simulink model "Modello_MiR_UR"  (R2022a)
settings: Solver=FixedStepAuto  StartTime=0.0  StopTime=time_s(end,1)  FixedStep=Sim.dt*10  RelTol=1e-3  EnableMultiTasking=on
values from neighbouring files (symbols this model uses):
  a = 0.250    (= 0.25)    [Modello_MiR_UR_script.m]    (also in Modello_MiR_2ruote_script.m; Modello_MiR_6ruote_script.m; Modello_MiR_6ruote_validato_script.m)
  a1 = 0.18265    [Modello_MiR_UR_script.m]    (also in UR_DHtable_e.m = 0; Modello_MiR_2ruote_script.m = deg2rad(5); Modello_MiR_6ruote_script.m = deg2rad(5); Modello_MiR_6ruote_validato_script.m)
  a2 = 0.40857    [Modello_MiR_UR_script.m]    (also in UR_DHtable_e.m = 612; Modello_MiR_2ruote_script.m = deg2rad(25); Modello_MiR_6ruote_script.m = deg2rad(25); Modello_MiR_6ruote_validato_script.m)
  Att_C1 = 0.01    [Modello_MiR_UR_script.m]    (also in Modello_MiR_6ruote_validato_script.m)
  Att_C2 = 0.01    [Modello_MiR_UR_script.m]    (also in Modello_MiR_6ruote_validato_script.m)
  Att_C5 = 0.01    [Modello_MiR_UR_script.m]    (also in Modello_MiR_6ruote_validato_script.m)
  Att_C6 = 0.01    [Modello_MiR_UR_script.m]    (also in Modello_MiR_6ruote_validato_script.m)
  b = 0.1875    [Modello_MiR_UR_script.m]    (also in Modello_MiR_2ruote_script.m; Modello_MiR_6ruote_script.m; Modello_MiR_6ruote_validato_script.m)
  b_caster = 0.07    [Modello_MiR_UR_script.m]    (also in Modello_MiR_2ruote_script.m; Modello_MiR_6ruote_script.m; Modello_MiR_6ruote_validato_script.m)
  bd = 0.205    [Modello_MiR_UR_script.m]    (also in Modello_MiR_2ruote_script.m; Modello_MiR_6ruote_script.m; Modello_MiR_6ruote_validato_script.m)
  F23MIR = @(u) (mv*9.801/4)-(mv*h*u(5)+(mv*9.801/4)*(2*a-b_caster*(cos(u(1))+cos(u(2)))))/(4*a-b_caster*(cos(u(1))+cos(u(2)))+b_caster*(cos(u(3))+cos(u(4))))    [Modello_MiR_UR_script.m]
  F23UR5 = @(u) (u(7)/4)-u(11)    [Modello_MiR_UR_script.m]
  F43MIR = @(u) (1/(2*bd))*(mv*u(6)*h+((mv*h*u(5)+(mv*9.801/4)*(2*a-b_caster*(cos(u(1))+cos(u(2)))))/(4*a-b_caster*(cos(u(1))+cos(u(2)))+b_caster*(cos(u(3))+cos(u(4)))))*(2*bd-b_caster*(sin(u(3))+sin(u(4))))+((mv*9.801/4)-(mv*h*u(5)+(mv*9.801/4)*(2*a-b_caster*(cos(u(1))+cos(u(2)))))/(4*a-b_caster*(cos(u(1))+cos(u(2)))+b_caster*(cos(u(3))+cos(u(4)))))*(2*bd-b_caster*(sin(u(1))+sin(u(2)))))    [Modello_MiR_UR_script.m]
  F43UR5 = @(u) (1/(2*bd))*(u(8) - u(6)*H +u(11)*(2*bd-b_caster*(sin(u(3))+sin(u(4))))+u(12)*(2*bd-b_caster*(sin(u(1))+sin(u(2)))))    [Modello_MiR_UR_script.m]
  F63MIR = @(u) (mv*h*u(5)+(mv*9.801/4)*(2*a-b_caster*(cos(u(1))+cos(u(2)))))/(4*a-b_caster*(cos(u(1))+cos(u(2)))+b_caster*(cos(u(3))+cos(u(4))))    [Modello_MiR_UR_script.m]
  F63UR5 = @(u)(-a*u(7)/2 -u(5)*H -u(9) +(u(7)/4)*(2*a-b_caster*(cos(u(1))+cos(u(2)))))/(4*a-b_caster*(cos(u(1))+cos(u(2)))+b_caster*(cos(u(3))+cos(u(4))))    [Modello_MiR_UR_script.m]
  f_c = 0.29564    [Modello_MiR_UR_script.m]    (also in Modello_MiR_6ruote_validato_script.m)
  f_d3 = 0.35846    [Modello_MiR_UR_script.m]    (also in Modello_MiR_6ruote_validato_script.m)
  f_d4 = 0.2333    [Modello_MiR_UR_script.m]    (also in Modello_MiR_6ruote_validato_script.m)
  fa_c = 0.27474    [Modello_MiR_UR_script.m]    (also in Modello_MiR_6ruote_validato_script.m)
  fa_d3 = 0.3694    [Modello_MiR_UR_script.m]    (also in Modello_MiR_6ruote_validato_script.m)
  fa_d4 = 0.28065    [Modello_MiR_UR_script.m]    (also in Modello_MiR_6ruote_validato_script.m)
  fm_fun = @(u) (u <= -am2 || u >= am2) * 0 + (u > -am2 && u <= -am1) * (- u* Mza/(am2 -am1) - Mza* am2/(am2 -am1)) +           + (u > -am1 && u <= am1) * (Mza * u / am1) + (u > am1 && u < am2) * (Mza * u /(am1 -am2) - Mza * am2 /(am1 - am2))    [Modello_MiR_UR_script.m]    (also in Modello_MiR_6ruote_script.m = @(u) (u <= -am2 | u >= am2)*0 + (u > -am2 && u <= -am1)*(- u; Modello_MiR_6ruote_validato_script.m)
  Hi = 1    [UR5e_data.m]
  Icw_1 = 1/2 * mcw * rc^2    (= 0.002004225735)    [Modello_MiR_UR_script.m]    (also in Modello_MiR_2ruote_script.m; Modello_MiR_6ruote_script.m; Modello_MiR_6ruote_validato_script.m)
  Icw_2 = 1/12 * mcw * ec^2 + 1/4 * mcw * rc^2    (= 0.00104098243873)    [Modello_MiR_UR_script.m]    (also in Modello_MiR_2ruote_script.m; Modello_MiR_6ruote_script.m; Modello_MiR_6ruote_validato_script.m)
  Idw_1 = 1/2 * mdw * rd^2    (= 0.00551836278784)    [Modello_MiR_UR_script.m]    (also in Modello_MiR_2ruote_script.m; Transfer_Function_Gol_Gcl.m = Inertia_vect(jj,1); Modello_MiR_6ruote_script.m; Modello_MiR_6ruote_validato_script.m)
  iMax = 20.7*1.1    (= 22.77)    [Modello_MiR_UR_script.m]    (also in Modello_MiR_2ruote_script.m; Modello_MiR_6ruote_script.m; Modello_MiR_6ruote_validato_script.m)
  Iv = mv * (l^2 + w^2)  / 12    (= 6.75343333333)    [Modello_MiR_UR_script.m]    (also in Modello_MiR_2ruote_script.m; Modello_MiR_6ruote_script.m; Modello_MiR_6ruote_validato_script.m = 8.95033333333)
  Kc = 0.15    [Modello_MiR_UR_script.m]    (also in Modello_MiR_2ruote_script.m; Modello_MiR_6ruote_script.m; Modello_MiR_6ruote_validato_script.m)
  Ki_i = 1    [Modello_MiR_UR_script.m]    (also in Modello_MiR_2ruote_script.m; Modello_MiR_6ruote_script.m; Modello_MiR_6ruote_validato_script.m)
  Ki_v = 1    [Modello_MiR_UR_script.m]    (also in Modello_MiR_2ruote_script.m; Modello_MiR_6ruote_script.m; Modello_MiR_6ruote_validato_script.m)
  kk = 0.00005    (= 5e-05)    [Modello_MiR_UR_script.m]    (also in Modello_MiR_2ruote_script.m; Modello_MiR_6ruote_script.m; Modello_MiR_6ruote_validato_script.m)
  Kp_i = 5    [Modello_MiR_UR_script.m]    (also in Modello_MiR_2ruote_script.m; Modello_MiR_6ruote_script.m; Modello_MiR_6ruote_validato_script.m)
  Kp_v = 5    [Modello_MiR_UR_script.m]    (also in Modello_MiR_2ruote_script.m; Modello_MiR_6ruote_script.m; Modello_MiR_6ruote_validato_script.m)
  kv = 1.5e-6    (= 1.5e-06)    [Modello_MiR_UR_script.m]    (also in Modello_MiR_2ruote_script.m; Modello_MiR_6ruote_script.m; Modello_MiR_6ruote_validato_script.m)
  L = R * tauE    (= 0.00181134822805)    [Modello_MiR_UR_script.m]    (also in Modello_MiR_2ruote_script.m; Modello_MiR_6ruote_script.m; Modello_MiR_6ruote_validato_script.m)
  mcw = rc^2 * pi * ec * rhopoliu + 1    (= 1.02616357632)    [Modello_MiR_UR_script.m]    (also in Modello_MiR_2ruote_script.m; Modello_MiR_6ruote_script.m; Modello_MiR_6ruote_validato_script.m)
  mv = 83    [Modello_MiR_UR_script.m]    (also in Modello_MiR_2ruote_script.m; Modello_MiR_6ruote_script.m; Modello_MiR_6ruote_validato_script.m = 110)
  Phi1_start = psi_mir(1,1)    [Modello_MiR_UR_script.m]    (also in Modello_MiR_6ruote_validato_script.m)
  Phi2_start = psi_mir(1,1)    [Modello_MiR_UR_script.m]    (also in Modello_MiR_6ruote_validato_script.m)
  Phi5_start = psi_mir(1,1)    [Modello_MiR_UR_script.m]    (also in Modello_MiR_6ruote_validato_script.m)
  Phi6_start = psi_mir(1,1)    [Modello_MiR_UR_script.m]    (also in Modello_MiR_6ruote_validato_script.m)
  Psi_start = psi_mir(1,1)    [Modello_MiR_UR_script.m]    (also in Modello_MiR_6ruote_script.m = 1.57079632679; Modello_MiR_6ruote_validato_script.m)
  q0 = [qset.q1.signals.values(1),qset.q2.signals.values(1),qset.q3.signals.values(1),qset.q4.signals.values(1),qset.q5.signals.values(1),qset.q6.signals.values(1)]    [UR5e_simmot.m]
  R = velMax * TorqueMax / (iMax)^2    (= 1.81134822805)    [Modello_MiR_UR_script.m]    (also in Modello_MiR_2ruote_script.m; Modello_MiR_6ruote_script.m; Modello_MiR_6ruote_validato_script.m)
  rap_rid = 10.167    [Modello_MiR_UR_script.m]    (also in Modello_MiR_2ruote_script.m; Modello_MiR_6ruote_script.m; Modello_MiR_6ruote_validato_script.m)
  rc = 0.125/2    (= 0.0625)    [Modello_MiR_UR_script.m]    (also in Modello_MiR_2ruote_script.m; Modello_MiR_6ruote_script.m; Modello_MiR_6ruote_validato_script.m)
  rd = 0.1    [Modello_MiR_UR_script.m]    (also in Modello_MiR_2ruote_script.m; Modello_MiR_6ruote_script.m; Modello_MiR_6ruote_validato_script.m)
  s = 1i*s    [Transfer_Function_Gol_Gcl.m]
  s1 = 0.18987    [Modello_MiR_UR_script.m]    (also in Modello_MiR_2ruote_script.m = 0.2; Modello_MiR_6ruote_script.m = 0.2; Modello_MiR_6ruote_validato_script.m)
  s2 = 0.99533    [Modello_MiR_UR_script.m]    (also in Modello_MiR_2ruote_script.m = 0.8; Modello_MiR_6ruote_script.m = 0.8; Modello_MiR_6ruote_validato_script.m)
  Sx = spline(x ,fl_fun(x),zx)    [Modello_MiR_6ruote_script.m]
  Sy = spline(x ,ft_fun(x),zy)    [Modello_MiR_6ruote_script.m]
  tau_i = 1/(2000*2*pi)    (= 7.95774715459e-05)    [UR5e_data.m]    (also in Transfer_Function_Gol_Gcl.m = Kp_i/Ki_i)
  VaMax = Kc * velMax    (= 41.2443991527)    [Modello_MiR_UR_script.m]    (also in Modello_MiR_2ruote_script.m; Modello_MiR_6ruote_script.m; Modello_MiR_6ruote_validato_script.m)
  X_start = traj(1,1)    [Modello_MiR_UR_script.m]    (also in Modello_MiR_2ruote_script.m = input('Inserire coordinata x iniziale'); Modello_MiR_6ruote_script.m = input('Inserire coordinata x iniziale'); Modello_MiR_6ruote_validato_script.m)
  Y_start = traj(1,2)    [Modello_MiR_UR_script.m]    (also in Modello_MiR_2ruote_script.m = input('Inserire coordinata y iniziale'); Modello_MiR_6ruote_script.m = input('Inserire coordinata y iniziale'); Modello_MiR_6ruote_validato_script.m)
undefined symbols (not defined in the file or in its folder): deg, Driver1, Driver2, Driver3, Driver4, Driver5, Driver6, Ground, J1, J2, J3, J4, J5, J6, kg, L1, L2, L3, L4, L5, L6, m, Motor, N, X, Y, z, Z
libraries: sm_lib x33, nesl_utility x30, slpidlib x10
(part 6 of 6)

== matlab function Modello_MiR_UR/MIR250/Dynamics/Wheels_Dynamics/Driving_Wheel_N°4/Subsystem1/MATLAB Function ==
function [Sx, z] = fcn(f, fa, s1, s2)
FLa =  fa  ;
FL = f  ;
Fx = @(u) (u <= -s2).* (-FL) + (u > -s2 & u <= -s1).*(u*(FL - FLa)/(s2 - s1) + s2*(FL - FLa)/(s2 - s1) - FL) +...
        + (u > -s1 & u <= s1).*(u * FLa / s1) + (u > s1 & u <= s2).* (u * (FLa - FL)/(s1 - s2) - s2 * (FLa - FL)/(s1 - s2) + FL) + ...
        + (u> s2) * FL;
% Interpolazione Cubica Attrito Longitudinale
nvet = 23 ; %specificare i numeri di nodi ( −1) della partizione
inferior = -1; % estremo inferiore intervallo
superi = 1 ; % estremo superiore intervallo
z = linspace(inferior,superi,10001); % definisco la griglia fine su cui valutare la spline
%figure
%set(gcf,'Position',[381 175 1208 753])

n = nvet ;
x = linspace(inferior, superi, n+1); % in questo esercizio definisco i nodi di interpolazione tra loro equispaziati
Sx = spline(x ,Fx(x),z) ; % valuto la spline cubica interpolante

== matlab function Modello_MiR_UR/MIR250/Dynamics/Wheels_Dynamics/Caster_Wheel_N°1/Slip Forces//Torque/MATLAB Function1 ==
function [Sy, z] = fcn(f, fa, a1, a2)
FTa = 1200/2500/0.6 * fa;
FT = 1200/2500/0.6 * f;
Fy_D = @(u) (u <= -a2).*(-FT) + (u > -a2 & u <= -a1).* (u*(FT - FTa)/(a2 - a1) + a2*(FT - FTa)/(a2 - a1) - FT) +...
+ (u > -a1 & u <= a1).* (u * FTa / a1) + (u > a1 & u <= a2).* (u * (FTa - FT)/(a1 - a2) - a2 * (FTa - FT)/(a1 - a2) + FT) + ...
+ (u > a2).* FT;

nvet = 20 ; %specificare i numeri di nodi ( −1) della partizione
inferior = -pi/2; % estremo inferiore intervallo
superi = pi/2 ; % estremo superiore intervallo
z = linspace(inferior,superi,10001); % definisco la griglia fine su cui valutare la spline

n = nvet ;
x = linspace(inferior, superi, n+1); % in questo esercizio definisco i nodi di interpolazione tra loro equispaziati
Sy = spline(x ,Fy_D(x),z) ; % valuto la spline cubica interpolante

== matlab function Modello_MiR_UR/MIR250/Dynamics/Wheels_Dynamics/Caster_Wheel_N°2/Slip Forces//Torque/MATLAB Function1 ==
function [Sy, z] = fcn(f, fa, a1, a2)
FTa = 1200/2500/0.6 * fa;
FT = 1200/2500/0.6 * f;
Fy_D = @(u) (u <= -a2).*(-FT) + (u > -a2 & u <= -a1).* (u*(FT - FTa)/(a2 - a1) + a2*(FT - FTa)/(a2 - a1) - FT) +...
+ (u > -a1 & u <= a1).* (u * FTa / a1) + (u > a1 & u <= a2).* (u * (FTa - FT)/(a1 - a2) - a2 * (FTa - FT)/(a1 - a2) + FT) + ...
+ (u > a2).* FT;

nvet = 20 ; %specificare i numeri di nodi ( −1) della partizione
inferior = -pi/2; % estremo inferiore intervallo
superi = pi/2 ; % estremo superiore intervallo
z = linspace(inferior,superi,10001); % definisco la griglia fine su cui valutare la spline

n = nvet ;
x = linspace(inferior, superi, n+1); % in questo esercizio definisco i nodi di interpolazione tra loro equispaziati
Sy = spline(x ,Fy_D(x),z) ; % valuto la spline cubica interpolante

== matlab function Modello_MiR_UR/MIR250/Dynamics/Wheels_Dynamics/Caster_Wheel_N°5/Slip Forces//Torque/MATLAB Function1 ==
function [Sy, z] = fcn(f, fa, a1, a2)
FTa = 1200/2500/0.6 * fa;
FT = 1200/2500/0.6 * f;
Fy_D = @(u) (u <= -a2).*(-FT) + (u > -a2 & u <= -a1).* (u*(FT - FTa)/(a2 - a1) + a2*(FT - FTa)/(a2 - a1) - FT) +...
+ (u > -a1 & u <= a1).* (u * FTa / a1) + (u > a1 & u <= a2).* (u * (FTa - FT)/(a1 - a2) - a2 * (FTa - FT)/(a1 - a2) + FT) + ...
+ (u > a2).* FT;

nvet = 20 ; %specificare i numeri di nodi ( −1) della partizione
inferior = -pi/2; % estremo inferiore intervallo
superi = pi/2 ; % estremo superiore intervallo
z = linspace(inferior,superi,10001); % definisco la griglia fine su cui valutare la spline

n = nvet ;
x = linspace(inferior, superi, n+1); % in questo esercizio definisco i nodi di interpolazione tra loro equispaziati
Sy = spline(x ,Fy_D(x),z) ; % valuto la spline cubica interpolante

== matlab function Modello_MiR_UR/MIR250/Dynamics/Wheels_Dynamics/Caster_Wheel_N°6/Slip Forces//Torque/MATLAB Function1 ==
function [Sy, z] = fcn(f, fa, a1, a2)
FTa = 1200/2500/0.6 * fa;
FT = 1200/2500/0.6 * f;
Fy_D = @(u) (u <= -a2).*(-FT) + (u > -a2 & u <= -a1).* (u*(FT - FTa)/(a2 - a1) + a2*(FT - FTa)/(a2 - a1) - FT) +...
+ (u > -a1 & u <= a1).* (u * FTa / a1) + (u > a1 & u <= a2).* (u * (FTa - FT)/(a1 - a2) - a2 * (FTa - FT)/(a1 - a2) + FT) + ...
+ (u > a2).* FT;

nvet = 20 ; %specificare i numeri di nodi ( −1) della partizione
inferior = -pi/2; % estremo inferiore intervallo
superi = pi/2 ; % estremo superiore intervallo
z = linspace(inferior,superi,10001); % definisco la griglia fine su cui valutare la spline

n = nvet ;
x = linspace(inferior, superi, n+1); % in questo esercizio definisco i nodi di interpolazione tra loro equispaziati
Sy = spline(x ,Fy_D(x),z) ; % valuto la spline cubica interpolante

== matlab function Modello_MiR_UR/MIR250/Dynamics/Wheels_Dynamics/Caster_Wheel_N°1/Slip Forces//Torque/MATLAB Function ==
function [Sx, z] = fcn(fc1, fac1, s1, s2)
f=fc1;
fa=fac1;
FLa =  fa  ;
FL = f  ;
Fx = @(u) (u <= -s2).* (-FL) + (u > -s2 & u <= -s1).*(u*(FL - FLa)/(s2 - s1) + s2*(FL - FLa)/(s2 - s1) - FL) +...
        + (u > -s1 & u <= s1).*(u * FLa / s1) + (u > s1 & u <= s2).* (u * (FLa - FL)/(s1 - s2) - s2 * (FLa - FL)/(s1 - s2) + FL) + ...
        + (u> s2) * FL;
% Interpolazione Cubica Attrito Longitudinale
nvet = 23 ; %specificare i numeri di nodi ( −1) della partizione
inferior = -1; % estremo inferiore intervallo
superi = 1 ; % estremo superiore intervallo
z = linspace(inferior,superi,10001); % definisco la griglia fine su cui valutare la spline
%figure
%set(gcf,'Position',[381 175 1208 753])

n = nvet ;
x = linspace(inferior, superi, n+1); % in questo esercizio definisco i nodi di interpolazione tra loro equispaziati
Sx = spline(x ,Fx(x),z) ; % valuto la spline cubica interpolante

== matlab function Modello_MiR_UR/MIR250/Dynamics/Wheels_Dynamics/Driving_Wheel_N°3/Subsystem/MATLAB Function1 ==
function [Sy, z] = fcn(f, fa, a1, a2)
FTa = 1200/2500/0.6 * fa;
FT = 1200/2500/0.6 * f;
Fy_D = @(u) (u <= -a2).*(-FT) + (u > -a2 & u <= -a1).* (u*(FT - FTa)/(a2 - a1) + a2*(FT - FTa)/(a2 - a1) - FT) +...
+ (u > -a1 & u <= a1).* (u * FTa / a1) + (u > a1 & u <= a2).* (u * (FTa - FT)/(a1 - a2) - a2 * (FTa - FT)/(a1 - a2) + FT) + ...
+ (u > a2).* FT;

nvet = 20 ; %specificare i numeri di nodi ( −1) della partizione
inferior = -pi/2; % estremo inferiore intervallo
superi = pi/2 ; % estremo superiore intervallo
z = linspace(inferior,superi,10001); % definisco la griglia fine su cui valutare la spline

n = nvet ;
x = linspace(inferior, superi, n+1); % in questo esercizio definisco i nodi di interpolazione tra loro equispaziati
Sy = spline(x ,Fy_D(x),z) ; % valuto la spline cubica interpolante

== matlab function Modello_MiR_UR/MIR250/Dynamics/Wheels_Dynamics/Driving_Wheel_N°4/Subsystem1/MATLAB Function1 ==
function [Sy, z] = fcn(f, fa, a1, a2)
FTa = 1200/2500/0.6 * fa;
FT = 1200/2500/0.6 * f;
Fy_D = @(u) (u <= -a2).*(-FT) + (u > -a2 & u <= -a1).* (u*(FT - FTa)/(a2 - a1) + a2*(FT - FTa)/(a2 - a1) - FT) +...
+ (u > -a1 & u <= a1).* (u * FTa / a1) + (u > a1 & u <= a2).* (u * (FTa - FT)/(a1 - a2) - a2 * (FTa - FT)/(a1 - a2) + FT) + ...
+ (u > a2).* FT;

nvet = 20 ; %specificare i numeri di nodi ( −1) della partizione
inferior = -pi/2; % estremo inferiore intervallo
superi = pi/2 ; % estremo superiore intervallo
z = linspace(inferior,superi,10001); % definisco la griglia fine su cui valutare la spline

n = nvet ;
x = linspace(inferior, superi, n+1); % in questo esercizio definisco i nodi di interpolazione tra loro equispaziati
Sy = spline(x ,Fy_D(x),z) ; % valuto la spline cubica interpolante

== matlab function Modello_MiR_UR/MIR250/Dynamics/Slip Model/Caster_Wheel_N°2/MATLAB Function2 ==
function Fc_neg_out = fcn(v_wheel,Vx_DL)
x=v_wheel;
y=Vx_DL;
cccc=1e20;

Fc_neg=@(x,y) ((((x-y)/abs(y+((1/cccc)*(y==0))))*(((x-y)/abs(y+((1/cccc)*(y==0))))>=-1)+ (-1)*(((x-y)/abs(y+((1/cccc)*(y==0))))<-1))*(x*y>=0 && y>=0) + (((x-y)/abs(x+((1/cccc)*(x==0))))*(((x-y)/abs(x+((1/cccc)*(x==0))))>=-1))*(x*y>0 && y<0) + (x*y<0)*(x/abs(x+((1/cccc)*(x==0)))) )*(0.02<(x^2+y^2)) +(10*(x-y)*(10*(x-y)>-1) -1*(10*(x-y)<=-1))*(0.02>=(x^2+y^2)); 
Fc_neg_out = Fc_neg(x,y);

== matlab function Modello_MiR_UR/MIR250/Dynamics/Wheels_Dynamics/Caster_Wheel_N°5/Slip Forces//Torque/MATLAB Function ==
function [Sx, z] = fcn(fc5, fac5, s1, s2)
f=fc5;
fa=fac5;
FLa =  fa  ;
FL = f  ;
Fx = @(u) (u <= -s2).* (-FL) + (u > -s2 & u <= -s1).*(u*(FL - FLa)/(s2 - s1) + s2*(FL - FLa)/(s2 - s1) - FL) +...
        + (u > -s1 & u <= s1).*(u * FLa / s1) + (u > s1 & u <= s2).* (u * (FLa - FL)/(s1 - s2) - s2 * (FLa - FL)/(s1 - s2) + FL) + ...
        + (u> s2) * FL;
% Interpolazione Cubica Attrito Longitudinale
nvet = 23 ; %specificare i numeri di nodi ( −1) della partizione
inferior = -1; % estremo inferiore intervallo
superi = 1 ; % estremo superiore intervallo
z = linspace(inferior,superi,10001); % definisco la griglia fine su cui valutare la spline
%figure
%set(gcf,'Position',[381 175 1208 753])

n = nvet ;
x = linspace(inferior, superi, n+1); % in questo esercizio definisco i nodi di interpolazione tra loro equispaziati
Sx = spline(x ,Fx(x),z) ; % valuto la spline cubica interpolante

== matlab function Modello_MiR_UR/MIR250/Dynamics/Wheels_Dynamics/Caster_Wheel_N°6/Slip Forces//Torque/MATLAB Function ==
function [Sx, z] = fcn(fc6, fac6, s1, s2)
f=fc6;
fa=fac6;
FLa =  fa  ;
FL = f  ;
Fx = @(u) (u <= -s2).* (-FL) + (u > -s2 & u <= -s1).*(u*(FL - FLa)/(s2 - s1) + s2*(FL - FLa)/(s2 - s1) - FL) +...
        + (u > -s1 & u <= s1).*(u * FLa / s1) + (u > s1 & u <= s2).* (u * (FLa - FL)/(s1 - s2) - s2 * (FLa - FL)/(s1 - s2) + FL) + ...
        + (u> s2) * FL;
% Interpolazione Cubica Attrito Longitudinale
nvet = 23 ; %specificare i numeri di nodi ( −1) della partizione
inferior = -1; % estremo inferiore intervallo
superi = 1 ; % estremo superiore intervallo
z = linspace(inferior,superi,10001); % definisco la griglia fine su cui valutare la spline
%figure
%set(gcf,'Position',[381 175 1208 753])

n = nvet ;
x = linspace(inferior, superi, n+1); % in questo esercizio definisco i nodi di interpolazione tra loro equispaziati
Sx = spline(x ,Fx(x),z) ; % valuto la spline cubica interpolante

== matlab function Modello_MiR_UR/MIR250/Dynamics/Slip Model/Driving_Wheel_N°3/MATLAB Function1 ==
function Fc_pos_out = fcn(v_wheel,Vx_DL)
x=v_wheel;
y=Vx_DL;
cccc=1e20;

Fc_pos=@(x,y) ((((x-y)/abs(x+((1/cccc)*(x==0))))*(((x-y)/abs(x+((1/cccc)*(x==0))))<=1 )+ 1*(((x-y)/abs(x+((1/cccc)*(x==0))))>1))*(x*y>=0 && x>=0) + (((x-y)/abs(y+((1/cccc)*(y==0))))*(((x-y)/abs(y+((1/cccc)*(y==0))))<=1 ))*(x*y>0 && x<0)+ (x*y<0)*(x/abs(x+((1/cccc)*(x==0)))))*(0.02<(x^2+y^2)) + (10*(x-y)*(10*(x-y)<1) +1*(10*(x-y)>=1))*(0.02>=(x^2+y^2));

Fc_pos_out = Fc_pos(x,y);

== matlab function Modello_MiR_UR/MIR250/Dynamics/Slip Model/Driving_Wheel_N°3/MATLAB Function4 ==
function Fc_neg_out = fcn(v_wheel,Vx_DL)

x=v_wheel;
y=Vx_DL;
cccc=1e20;

Fc_neg=@(x,y) ((((x-y)/abs(y+((1/cccc)*(y==0))))*(((x-y)/abs(y+((1/cccc)*(y==0))))>=-1)+ (-1)*(((x-y)/abs(y+((1/cccc)*(y==0))))<-1))*(x*y>=0 && y>=0) + (((x-y)/abs(x+((1/cccc)*(x==0))))*(((x-y)/abs(x+((1/cccc)*(x==0))))>=-1))*(x*y>0 && y<0) + (x*y<0)*(x/abs(x+((1/cccc)*(x==0)))) )*(0.02<(x^2+y^2)) +(10*(x-y)*(10*(x-y)>-1) -1*(10*(x-y)<=-1))*(0.02>=(x^2+y^2)); 
Fc_neg_out = Fc_neg(x,y);

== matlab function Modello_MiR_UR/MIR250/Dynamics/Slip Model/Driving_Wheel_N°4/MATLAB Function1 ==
function Fc_pos_out = fcn(v_wheel,Vx_DL)
x=v_wheel;
y=Vx_DL;
cccc=1e20;

Fc_pos=@(x,y) ((((x-y)/abs(x+((1/cccc)*(x==0))))*(((x-y)/abs(x+((1/cccc)*(x==0))))<=1 )+ 1*(((x-y)/abs(x+((1/cccc)*(x==0))))>1))*(x*y>=0 && x>=0) + (((x-y)/abs(y+((1/cccc)*(y==0))))*(((x-y)/abs(y+((1/cccc)*(y==0))))<=1 ))*(x*y>0 && x<0)+ (x*y<0)*(x/abs(x+((1/cccc)*(x==0)))))*(0.02<(x^2+y^2)) + (10*(x-y)*(10*(x-y)<1) +1*(10*(x-y)>=1))*(0.02>=(x^2+y^2));

Fc_pos_out = Fc_pos(x,y);

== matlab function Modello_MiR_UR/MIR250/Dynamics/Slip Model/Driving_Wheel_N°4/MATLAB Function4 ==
function Fc_neg_out = fcn(v_wheel,Vx_DL)
x=v_wheel;
y=Vx_DL;
cccc=1e20;

Fc_neg=@(x,y) ((((x-y)/abs(y+((1/cccc)*(y==0))))*(((x-y)/abs(y+((1/cccc)*(y==0))))>=-1)+ (-1)*(((x-y)/abs(y+((1/cccc)*(y==0))))<-1))*(x*y>=0 && y>=0) + (((x-y)/abs(x+((1/cccc)*(x==0))))*(((x-y)/abs(x+((1/cccc)*(x==0))))>=-1))*(x*y>0 && y<0) + (x*y<0)*(x/abs(x+((1/cccc)*(x==0)))) )*(0.02<(x^2+y^2)) +(10*(x-y)*(10*(x-y)>-1) -1*(10*(x-y)<=-1))*(0.02>=(x^2+y^2)); 
Fc_neg_out = Fc_neg(x,y);

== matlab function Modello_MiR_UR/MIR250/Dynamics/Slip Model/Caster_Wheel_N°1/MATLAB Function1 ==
function Fc_pos_out = fcn(v_wheel,Vx_DL)
x=v_wheel;
y=Vx_DL;
cccc=1e20;

Fc_pos=@(x,y) ((((x-y)/abs(x+((1/cccc)*(x==0))))*(((x-y)/abs(x+((1/cccc)*(x==0))))<=1 )+ 1*(((x-y)/abs(x+((1/cccc)*(x==0))))>1))*(x*y>=0 && x>=0) + (((x-y)/abs(y+((1/cccc)*(y==0))))*(((x-y)/abs(y+((1/cccc)*(y==0))))<=1 ))*(x*y>0 && x<0)+ (x*y<0)*(x/abs(x+((1/cccc)*(x==0)))))*(0.02<(x^2+y^2)) + (10*(x-y)*(10*(x-y)<1) +1*(10*(x-y)>=1))*(0.02>=(x^2+y^2));

Fc_pos_out = Fc_pos(x,y);

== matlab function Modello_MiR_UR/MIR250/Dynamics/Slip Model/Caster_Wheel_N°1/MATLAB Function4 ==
function Fc_neg_out = fcn(v_wheel,Vx_DL)
x=v_wheel;
y=Vx_DL;
cccc=1e20;

Fc_neg=@(x,y) ((((x-y)/abs(y+((1/cccc)*(y==0))))*(((x-y)/abs(y+((1/cccc)*(y==0))))>=-1)+ (-1)*(((x-y)/abs(y+((1/cccc)*(y==0))))<-1))*(x*y>=0 && y>=0) + (((x-y)/abs(x+((1/cccc)*(x==0))))*(((x-y)/abs(x+((1/cccc)*(x==0))))>=-1))*(x*y>0 && y<0) + (x*y<0)*(x/abs(x+((1/cccc)*(x==0)))) )*(0.02<(x^2+y^2)) +(10*(x-y)*(10*(x-y)>-1) -1*(10*(x-y)<=-1))*(0.02>=(x^2+y^2)); 
Fc_neg_out = Fc_neg(x,y);
